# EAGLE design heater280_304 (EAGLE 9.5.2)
DATABASE: Z:\Eigene Dateien\Anwendungsdaten\Eagle\partdb\exp.txt
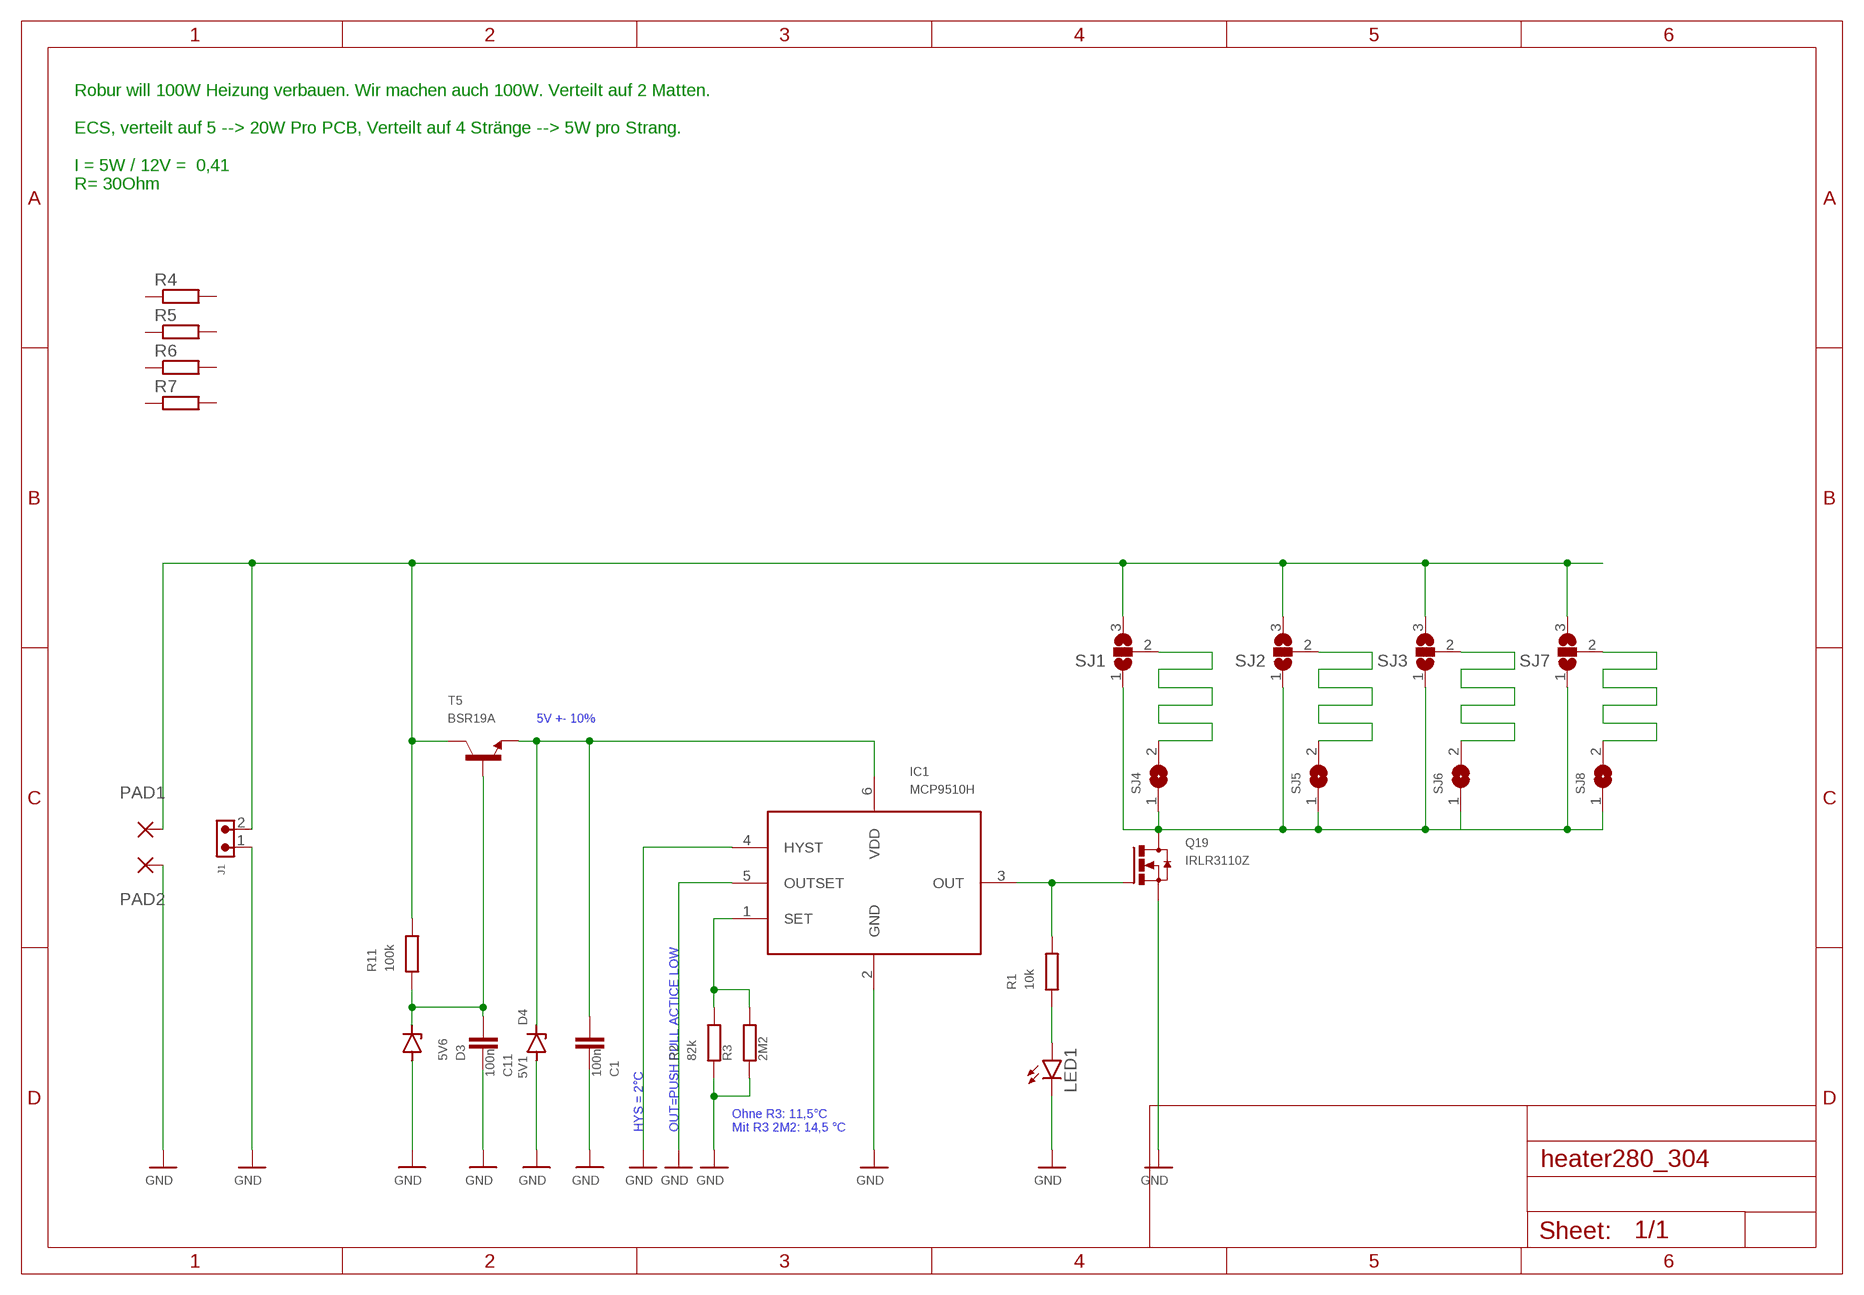
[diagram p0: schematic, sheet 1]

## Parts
C1  100n  C-EUC0603  [C0603]
C11  100n  C-EUC0603  [C0603]
D3  5V6  ZENER-DIODESOD80C  [SOD80C]
D4  5V1  ZENER-DIODESOD80C  [SOD80C]
IC1  MCP9510H  MCP9509  [SOT23-6]
J1  691322110002  [691322110002]
LED1  LEDSML0603  [SML0603]
PAD1  3,81/1,4  [3,81/1,4]
PAD2  3,81/1,4  [3,81/1,4]
Q19  IRLR3110Z  IRFR2607  [D-PACK]
R1  10k  R-EU_R0603  [R0603]
R2  82k  R-EU_R0603  [R0603]
R3  2M2  R-EU_R0603  [R0603]
R4  R-EU_R1206  [R1206]
R5  R-EU_R1206  [R1206]
R6  R-EU_R1206  [R1206]
R7  R-EU_R1206  [R1206]
R11  100k  R-EU_R0603  [R0603]
SJ1  SJ2W  [SJ_2]
SJ2  SJ2W  [SJ_2]
SJ3  SJ2W  [SJ_2]
SJ4  SJ  [SJ]
SJ5  SJ  [SJ]
SJ6  SJ  [SJ]
SJ7  SJ2W  [SJ_2]
SJ8  SJ  [SJ]
T5  BSR19A  MMBT2222ALT1-NPN-SOT23-BEC  [SOT23-BEC]

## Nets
+UB: J1.2 PAD1.1(P) R11.2 SJ1.3 SJ2.3 SJ3.3 SJ7.3 T5.C
GND: C1.2 C11.2 D3.A D4.A IC1.2(GND) IC1.4(HYST) IC1.5(OUTSET) J1.1 LED1.C PAD2.1(P) Q19.3(S) R2.1 R3.1
N$1: IC1.3(OUT) Q19.1(G) R1.2
N$2: SJ1.2 SJ4.2
N$3: C11.1 D3.C R11.1 T5.B
N$4: IC1.1(SET) R2.2 R3.2
N$5: C1.1 D4.C IC1.6(VDD) T5.E
N$6: LED1.A R1.1
N$7: SJ2.2 SJ5.2
N$8: SJ3.2 SJ6.2
N$9: SJ7.2 SJ8.2
N$11: Q19.4(D) SJ1.1 SJ2.1 SJ3.1 SJ4.1 SJ5.1 SJ6.1 SJ7.1 SJ8.1
Unconnected: R4.1 R4.2 R5.1 R5.2 R6.1 R6.2 R7.1 R7.2

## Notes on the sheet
- Robur will 100W Heizung verbauen. Wir machen auch 100W. Verteilt auf 2 Matten.
  
  ECS, verteilt auf 5 --> 20W Pro PCB, Verteilt auf 4 Stränge --> 5W pro Strang.
  
  I = 5W / 12V =  0,41
  R= 30Ohm
- 5V +- 10%
- HYS = 2°C | OUT=PUSH PULL ACTICE LOW
- Ohne R3: 11,5°C
  Mit R3 2M2: 14,5 °C

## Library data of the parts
C1 C11 = rcl:C-EU: CAPACITOR, European symbol; PARTNO: C067; SPICEPREFIX: C
D3 = diode:ZENER-DIODE: Z-Diode; PARTNO: D013
D4 = diode:ZENER-DIODE: Z-Diode; PARTNO: D012
IC1 = mcp9509:MCP9509; PARTNO: IC333
J1 = Wurth_Connectors_WR-TBL Pluggable Connector:691322110002: WR-TBL Serie 3221 - 3.50 mm Horizontal PCB Header; DATASHEET-URL: https://www.we-online.com/catalog/datasheet/691322110002.pdf; IR-UL: 10A; IR-VDE: 10.5A; MOUNT: THT; PART-NUMBER: 691322110002; PARTNO: CON212; PINS: 2; PITCH: 3.5mm; TYPE: Horizontal; WORKING-VOLTAGE-UL: 300V (AC); WORKING-VOLTAGE-VDE: 300V (AC)
LED1 = led:LED: LED; PARTNO: D078
PAD1 PAD2 = wirepad:3,81/1,4: THROUGH-HOLE PAD
Q19 = IRFR2607:IRFR2607; PARTNO: T086
R1 = rcl:R-EU_: RESISTOR, European symbol; PARTNO: R221; SPICEPREFIX: R
R2 = rcl:R-EU_: RESISTOR, European symbol; PARTNO: R243; SPICEPREFIX: R
R3 R11 = rcl:R-EU_: RESISTOR, European symbol; PARTNO: R245; SPICEPREFIX: R
R4-R7 = rcl:R-EU_: RESISTOR, European symbol; PARTNO: R493; SPICEPREFIX: R
SJ1-SJ3 SJ7 = jumper:SJ2W: SMD solder JUMPER
SJ4-SJ6 SJ8 = jumper:SJ: SMD solder JUMPER
T5 = transistor-neu-to92:*-NPN-: NPN Transistror; PARTNO: T056

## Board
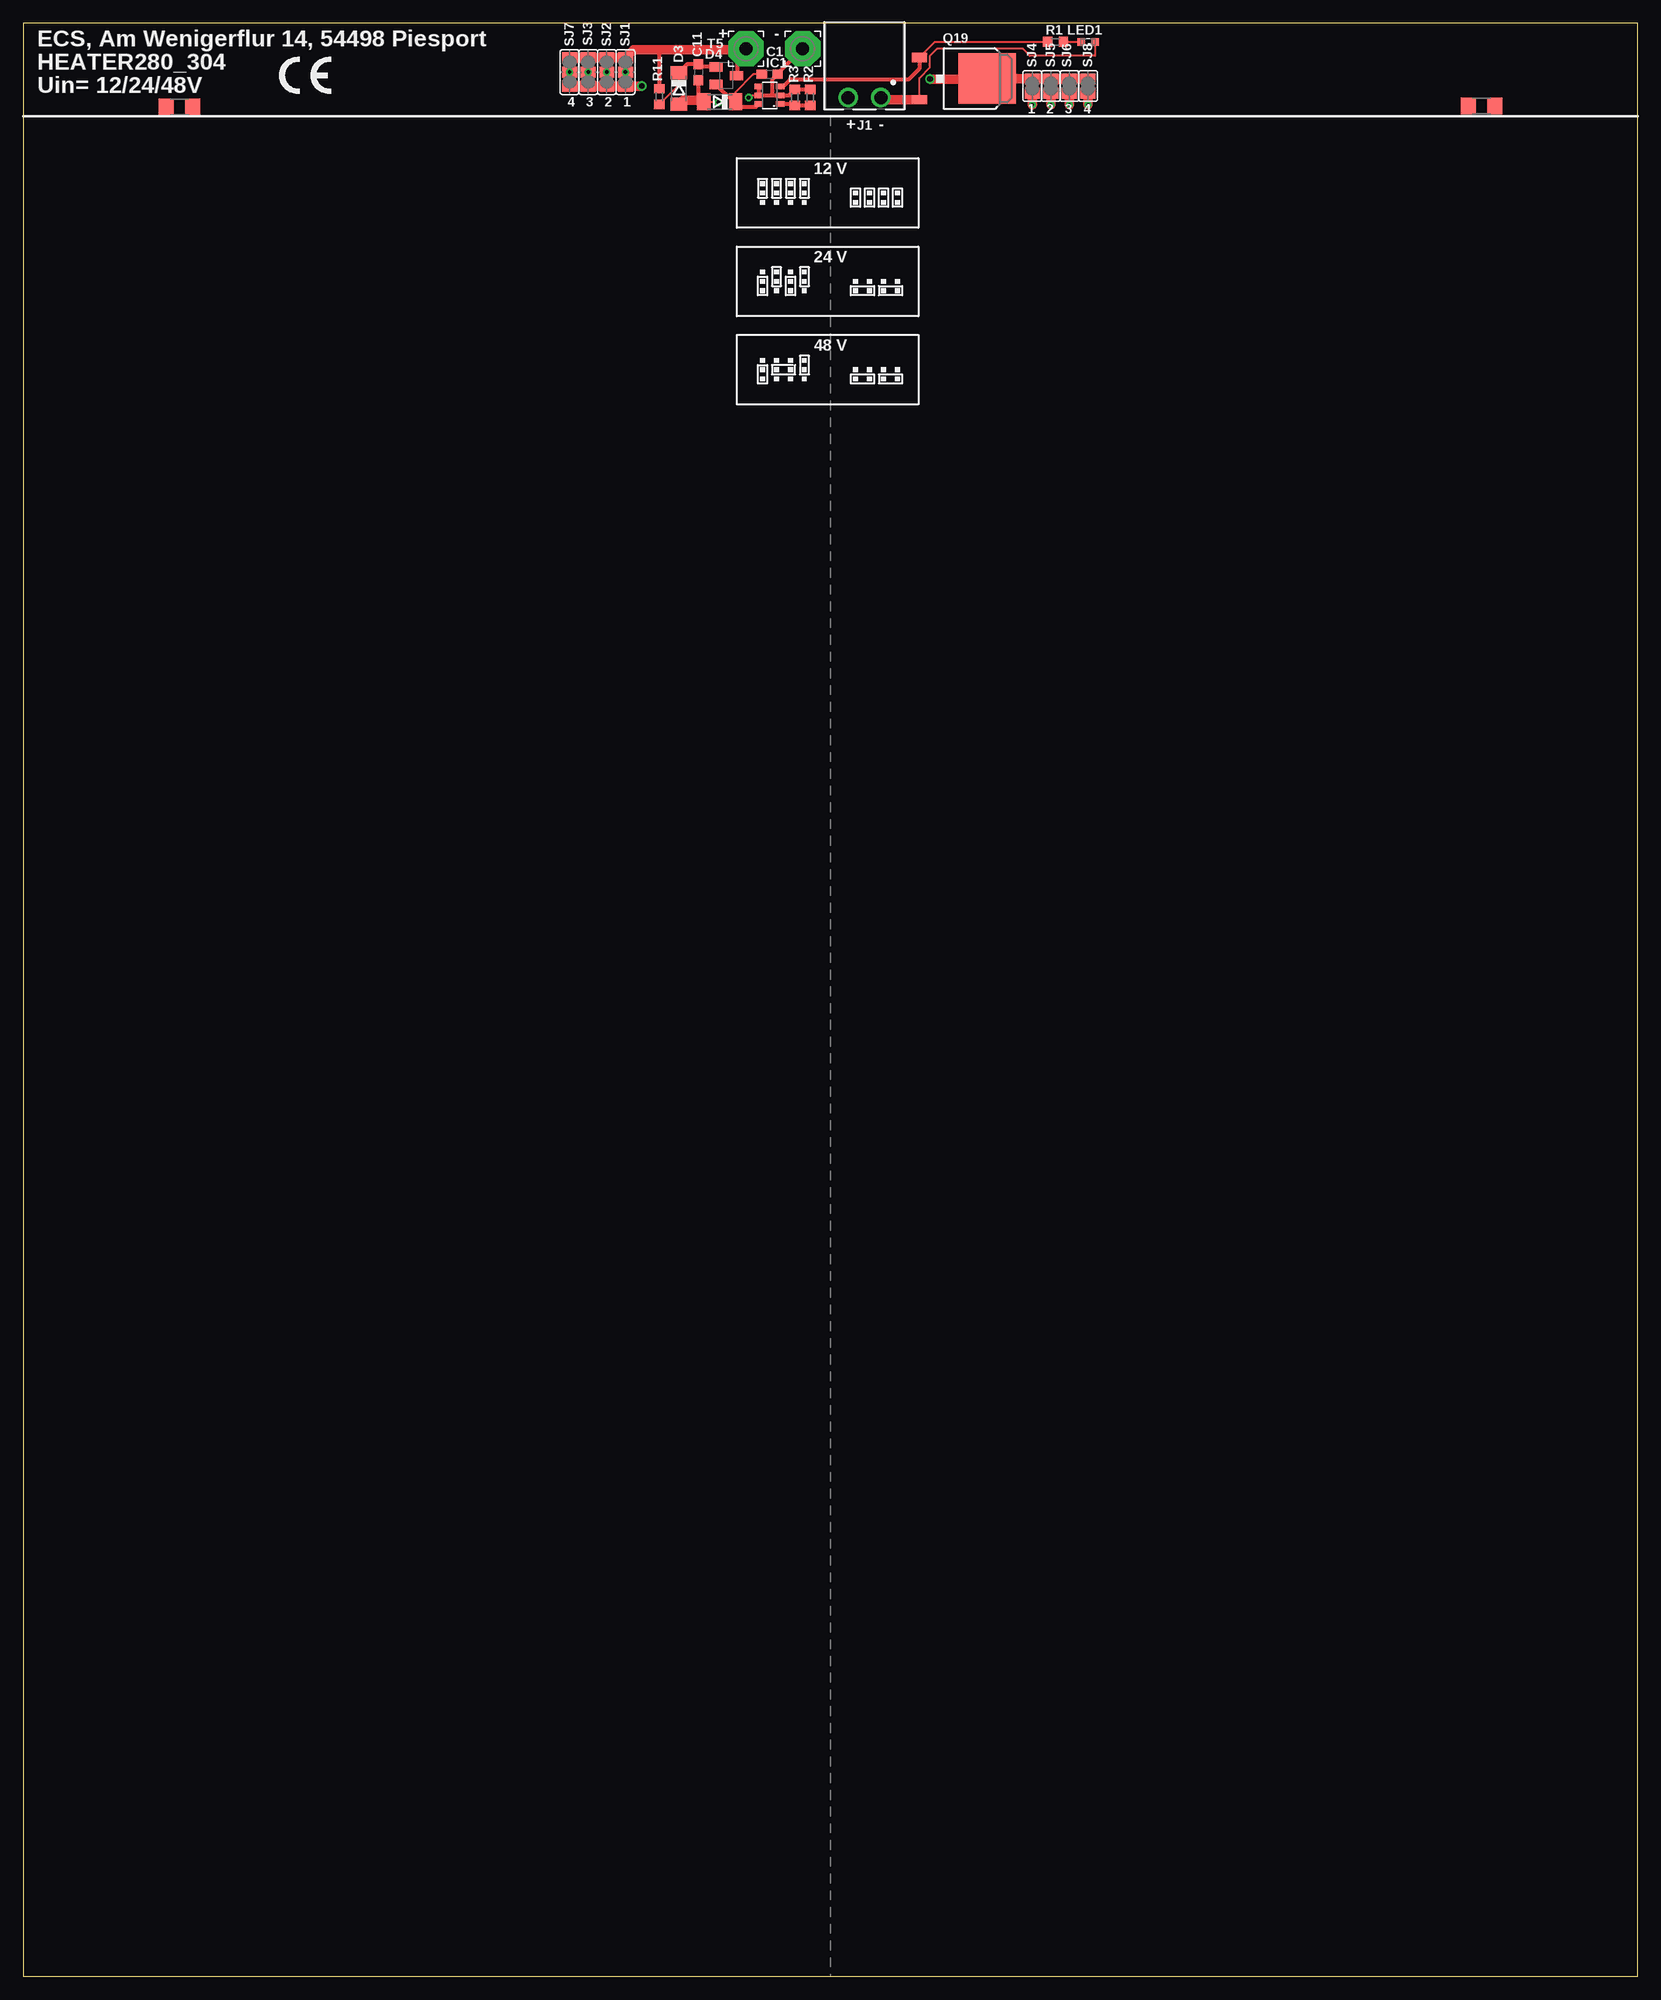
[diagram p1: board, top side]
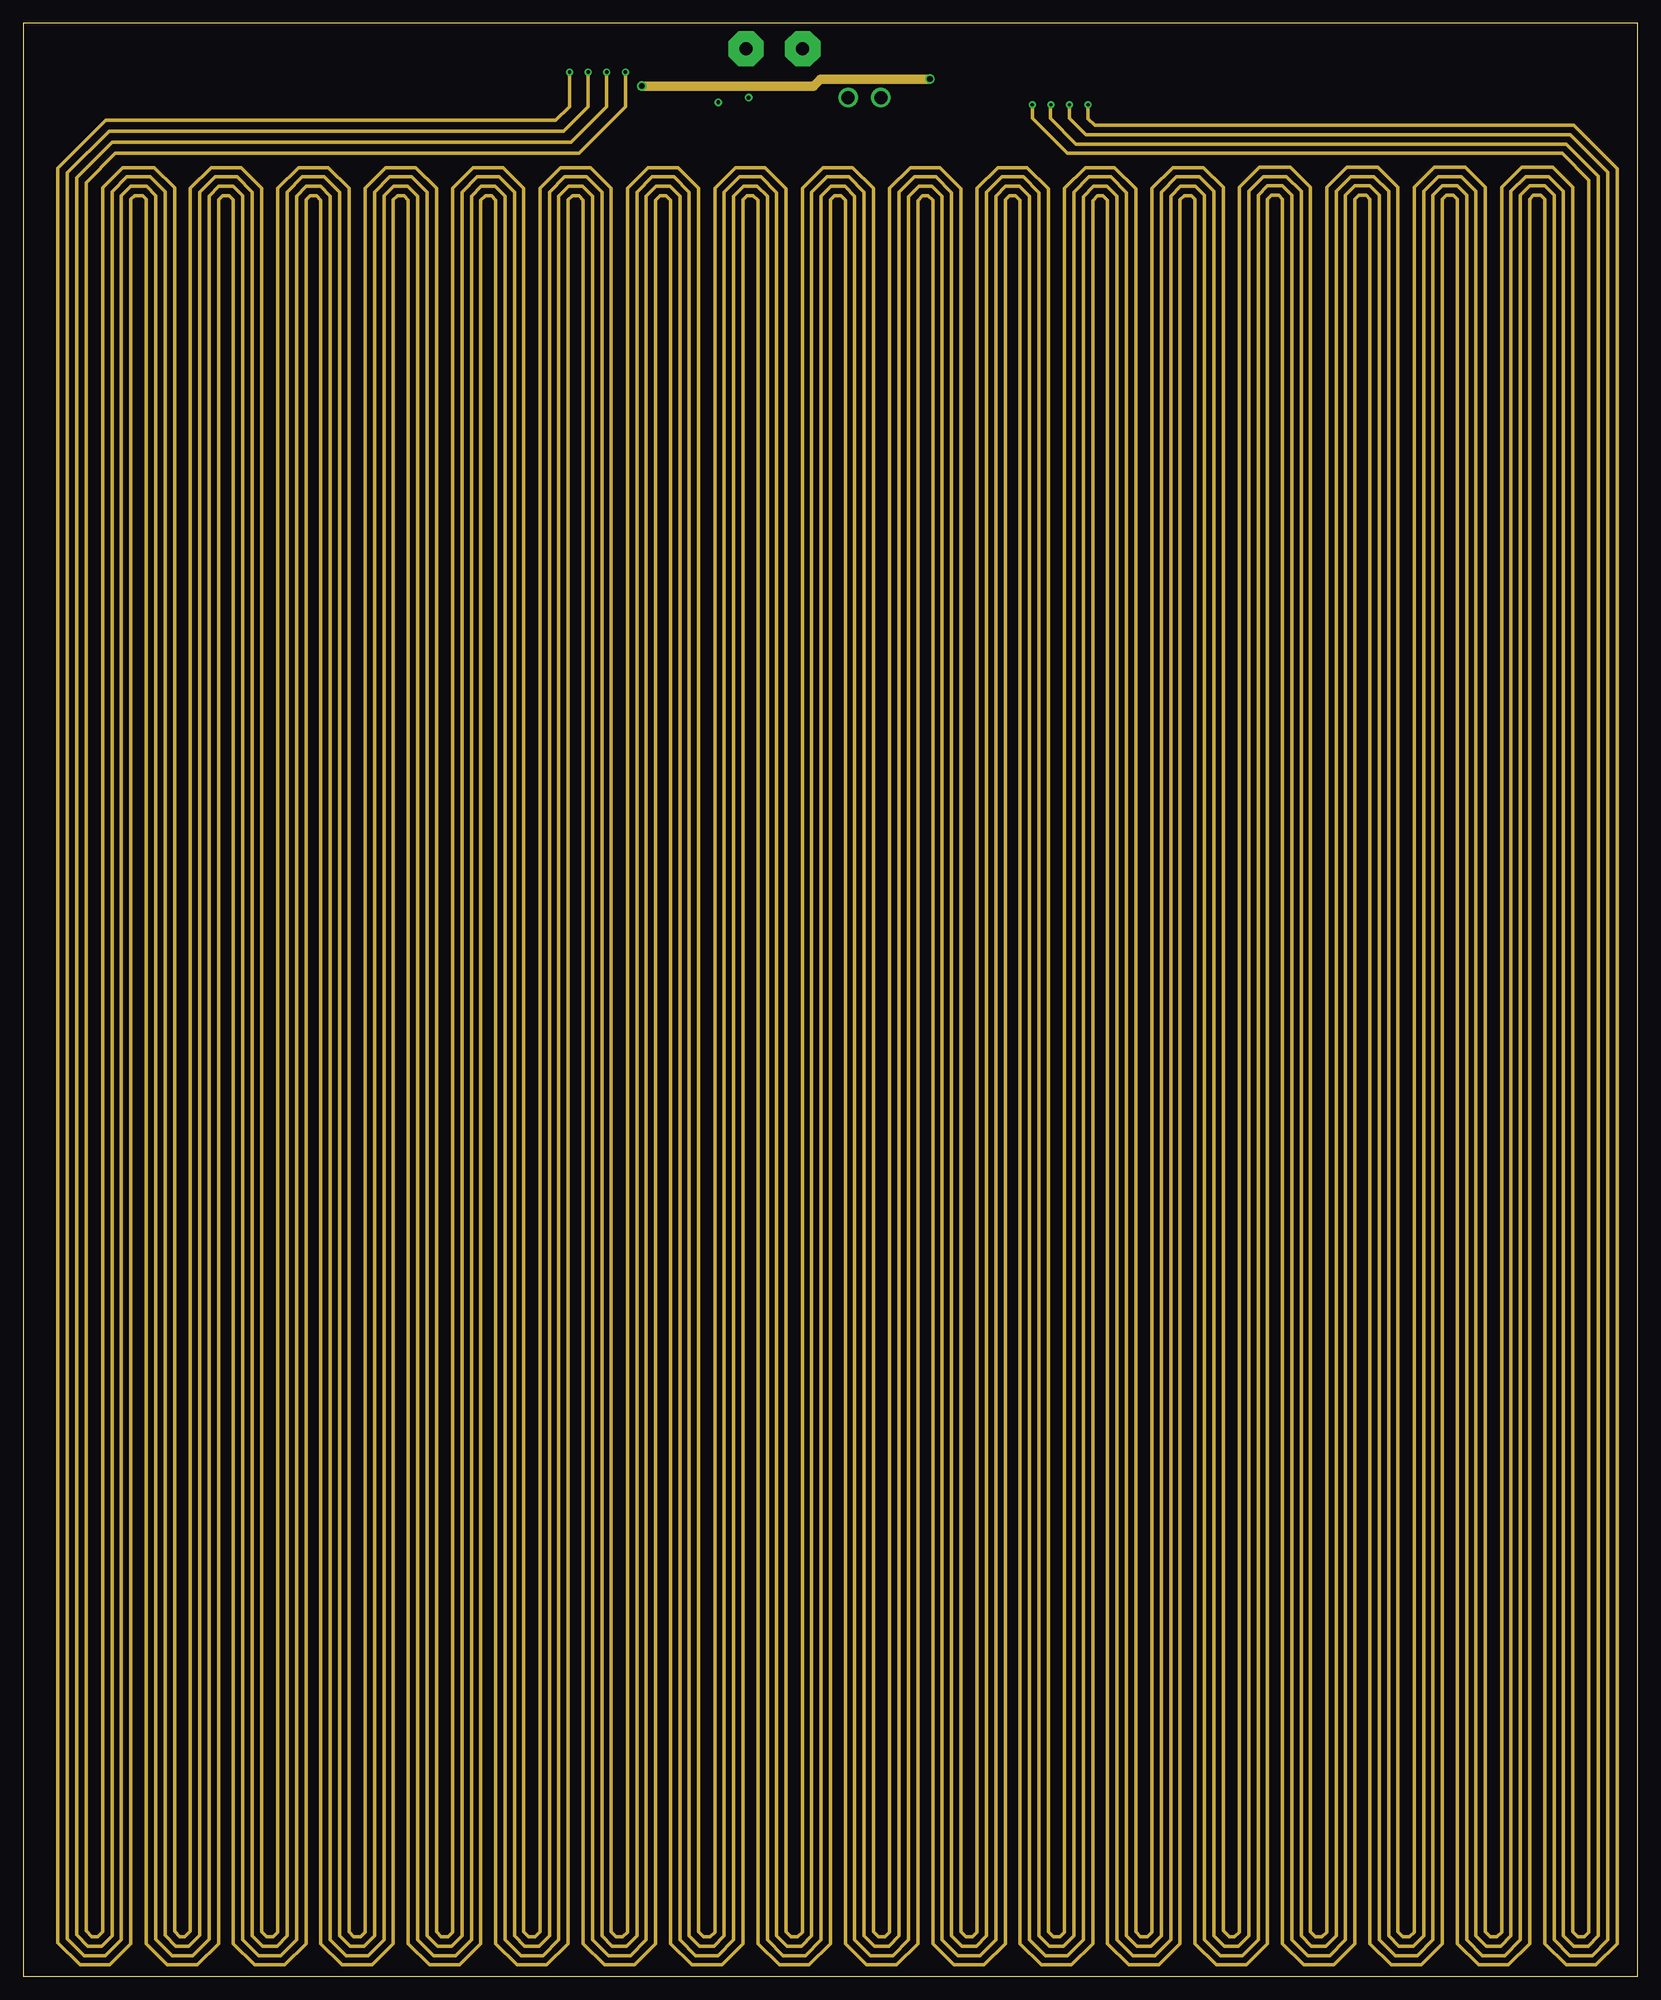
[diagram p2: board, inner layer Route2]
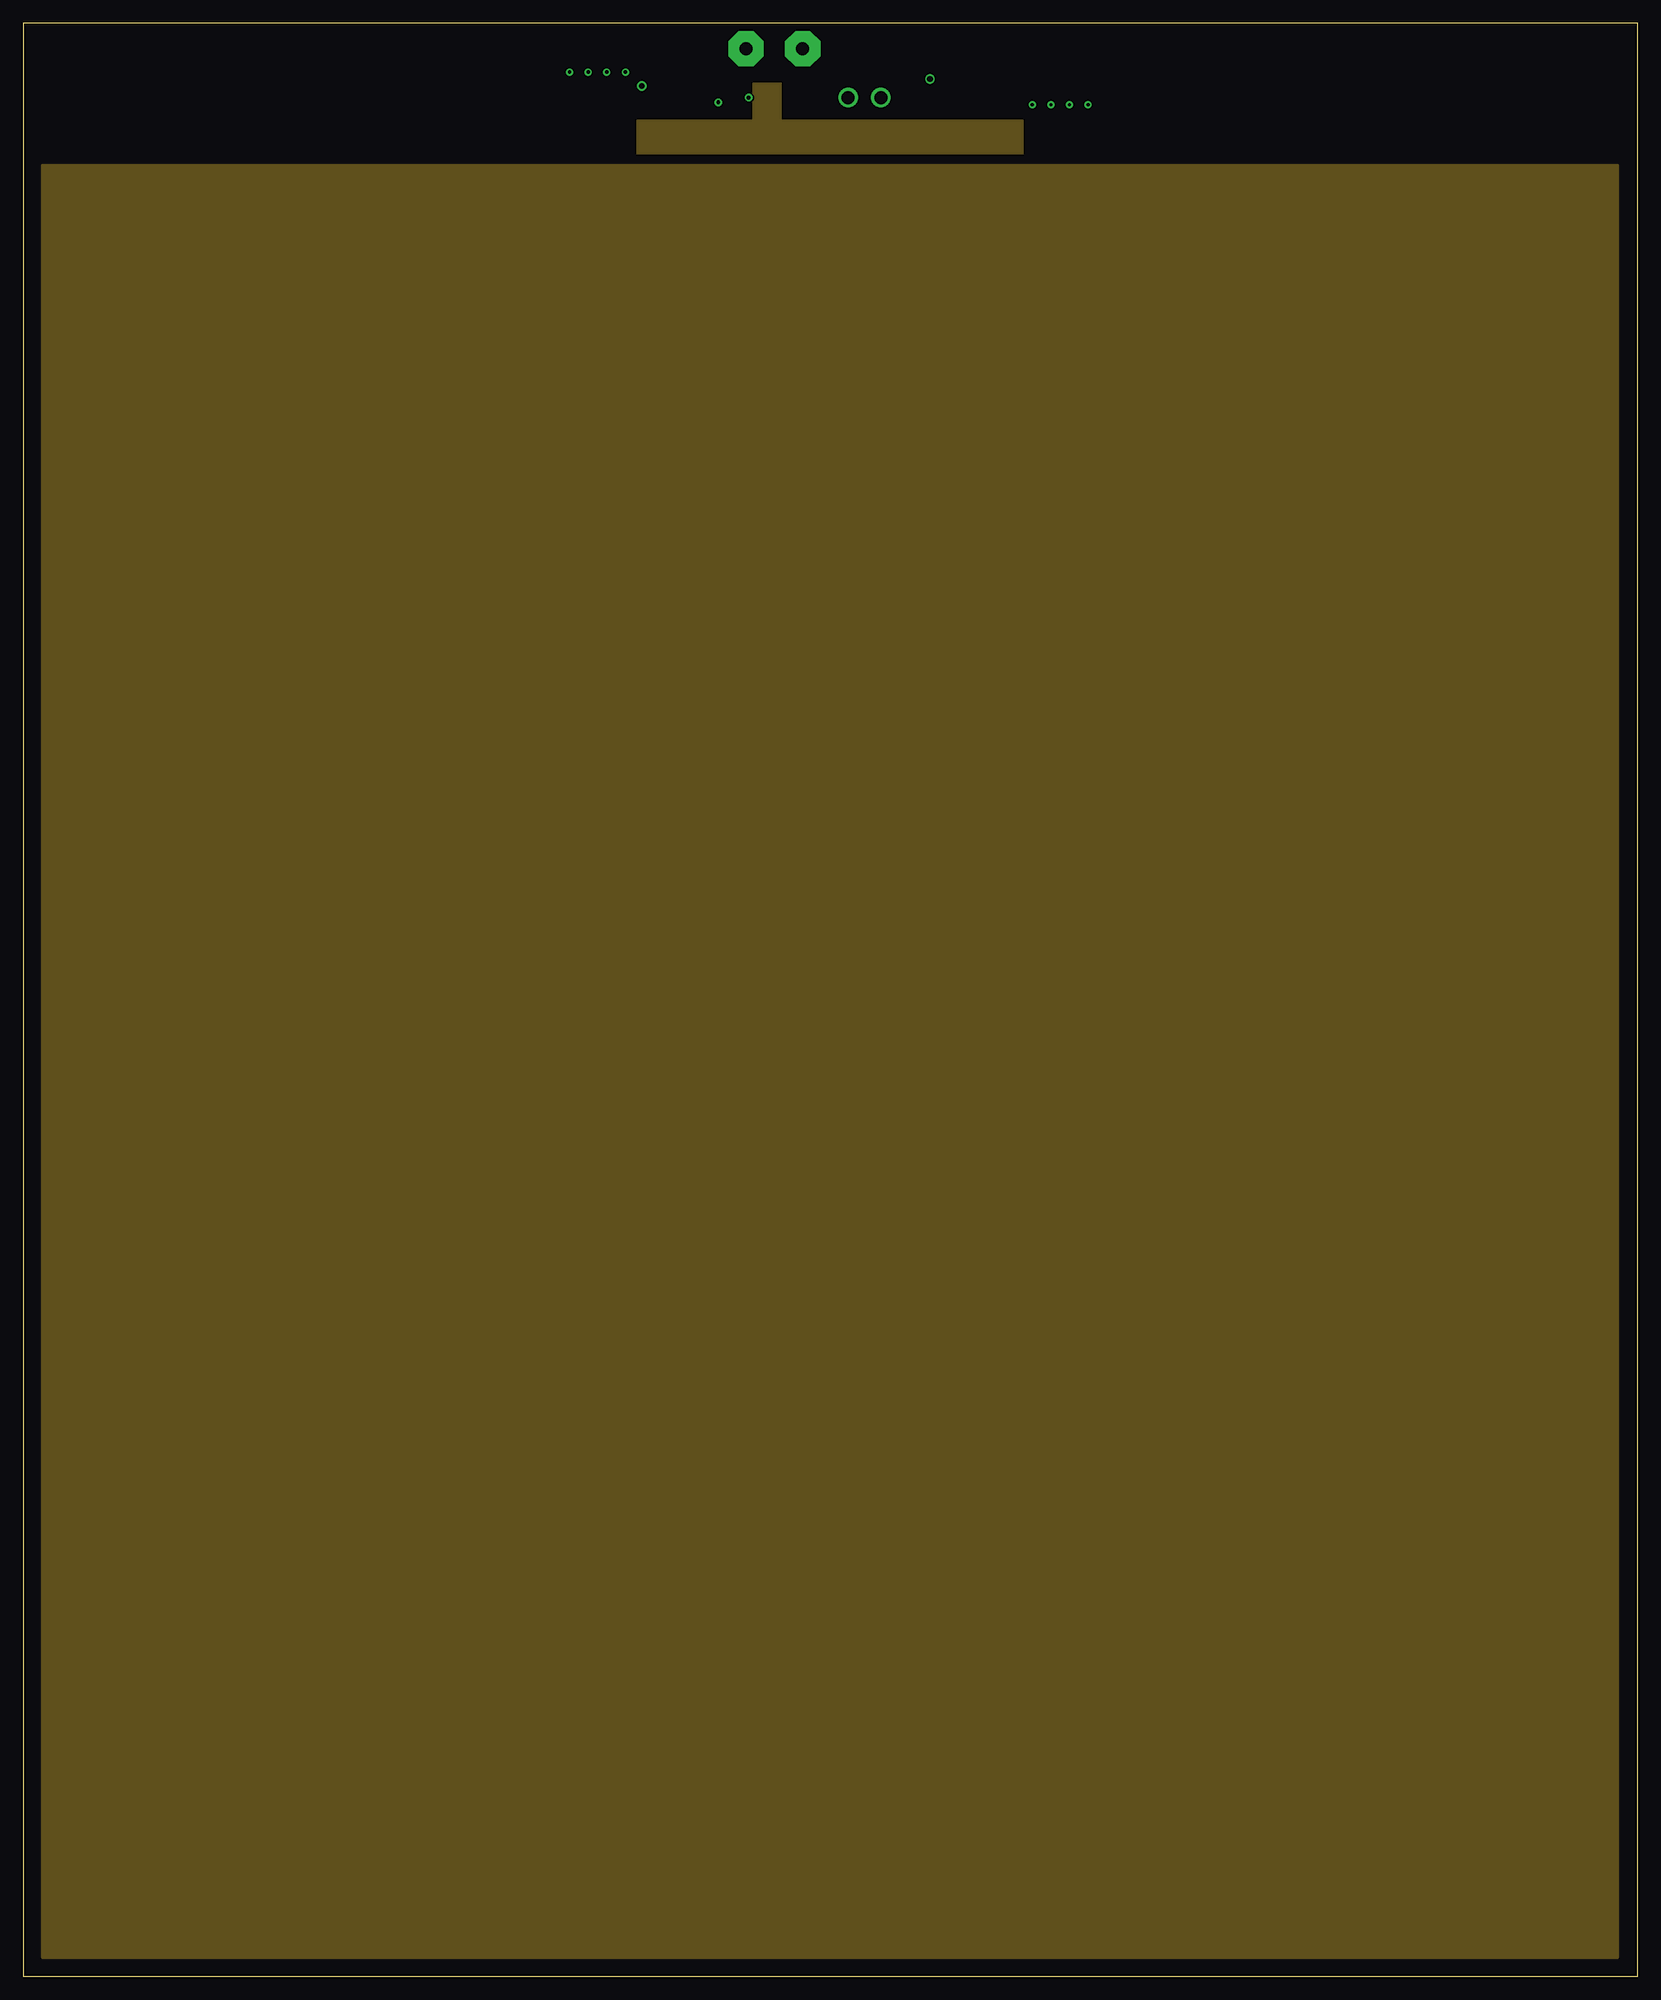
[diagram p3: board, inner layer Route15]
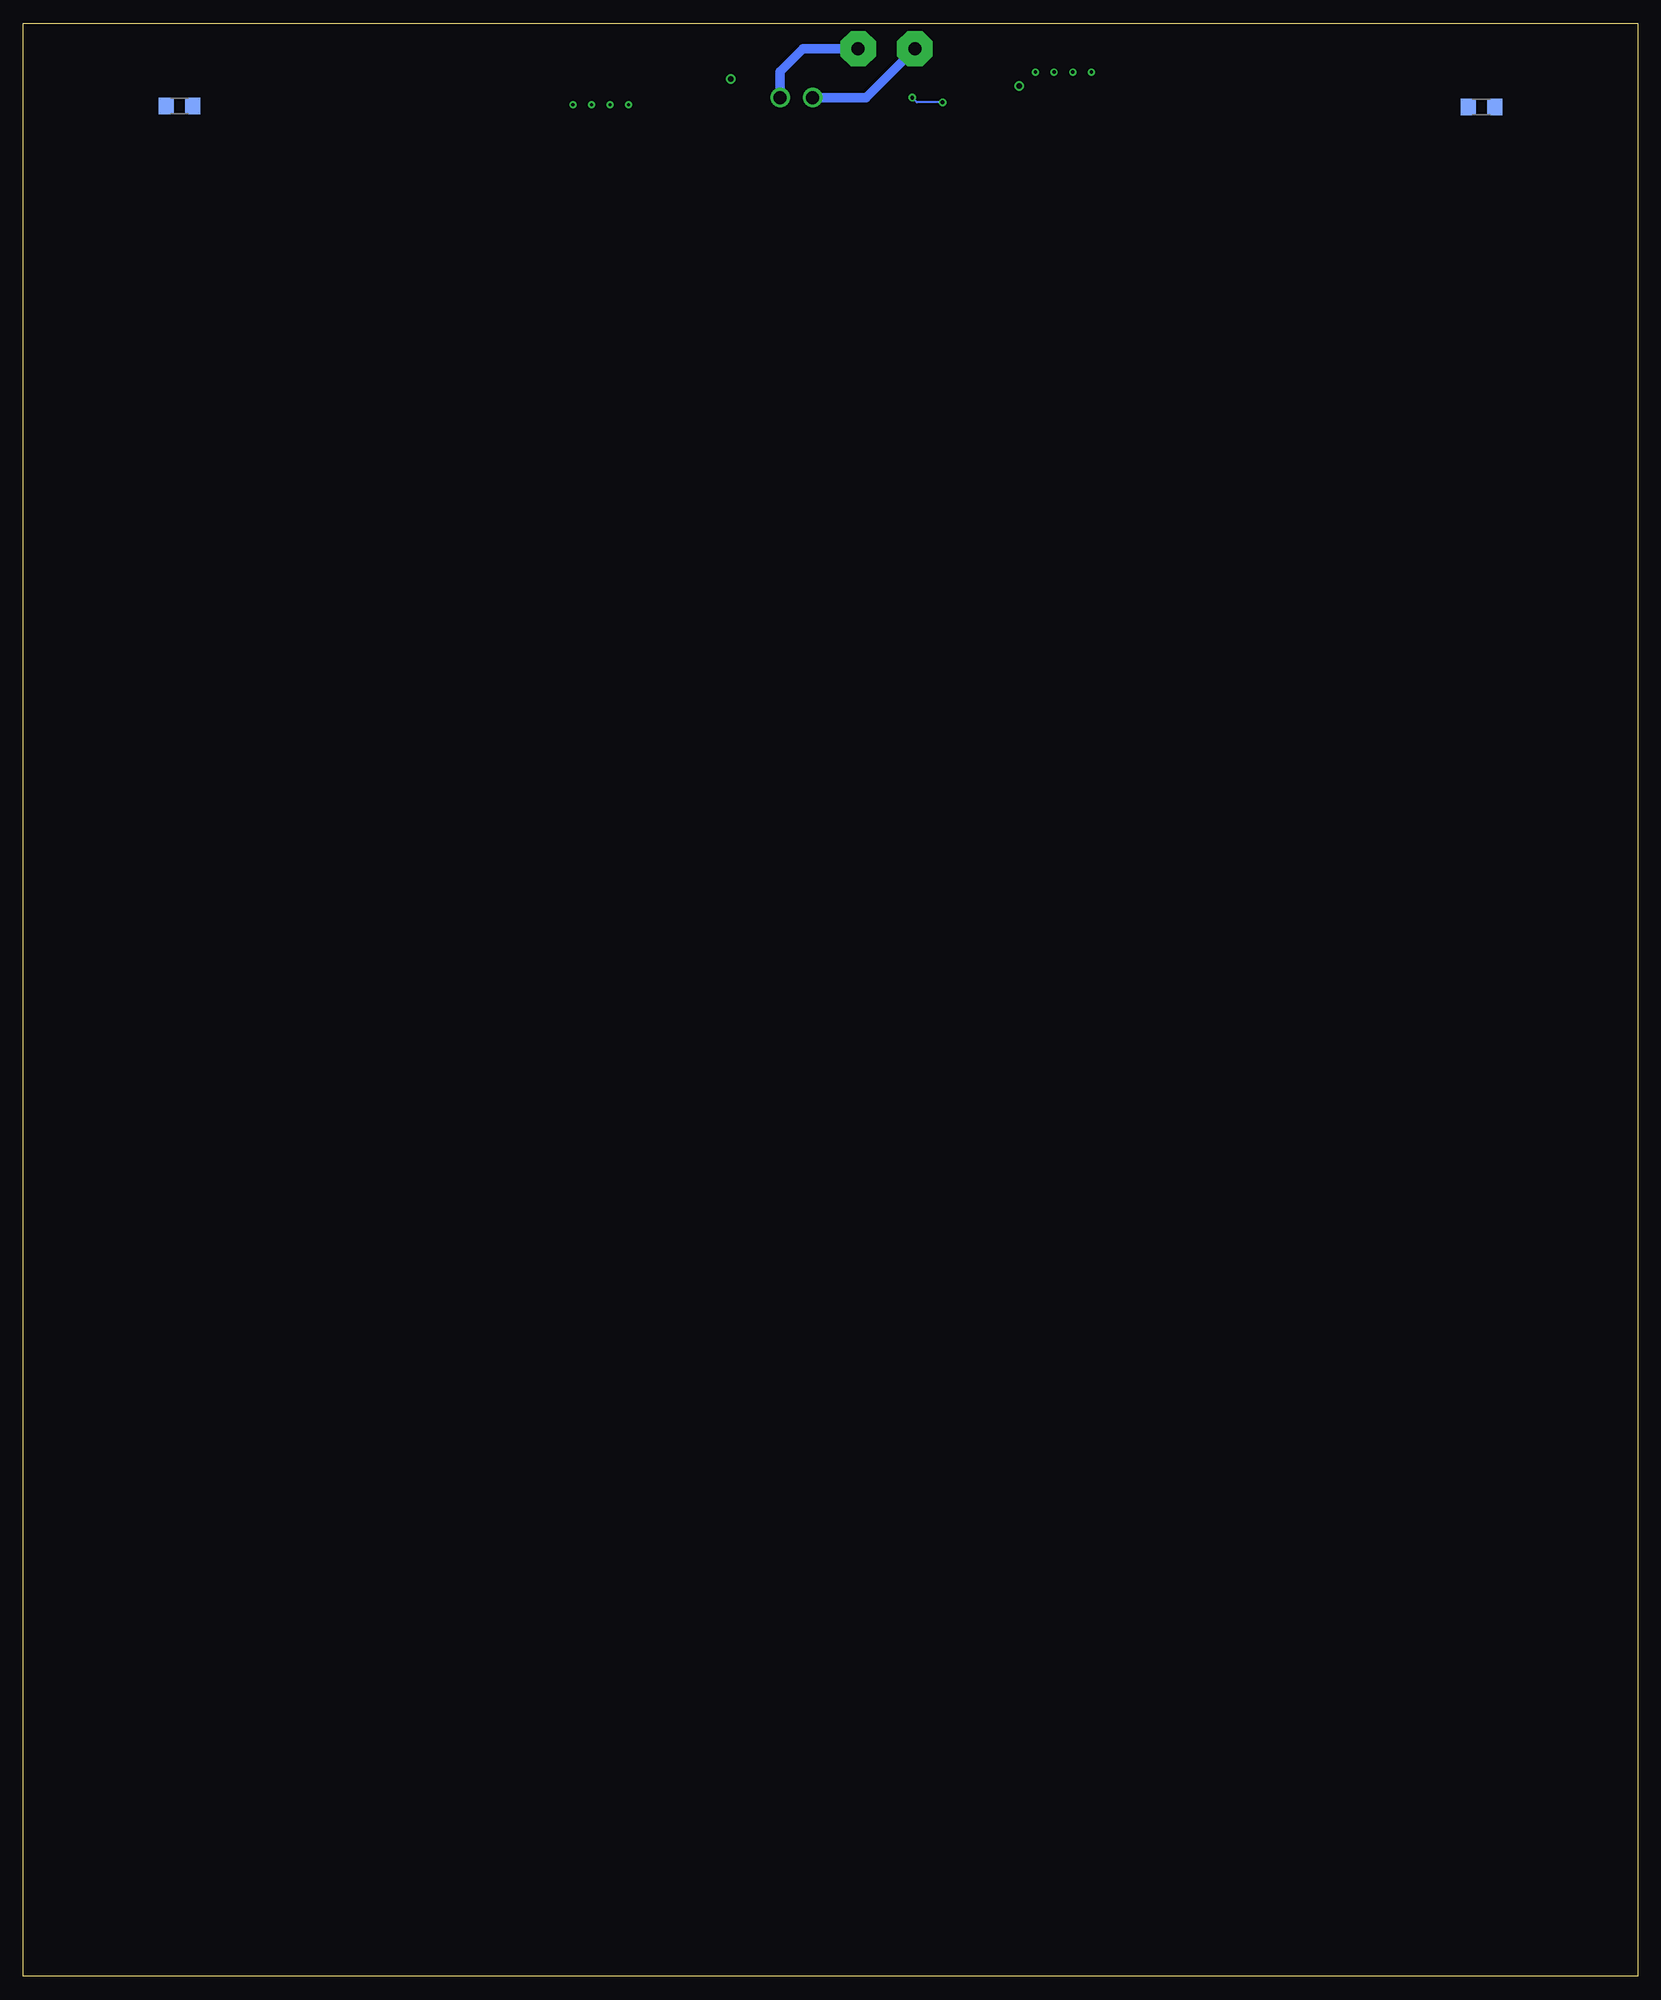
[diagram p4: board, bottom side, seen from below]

Size 173.6 x 210 mm. Coordinates in mm from the lower left corner, seen from the top.
Outline: 0,0 173.6,0 173.6,210 0,210 0,0
Copper layers (1+2*15+16): Top 0.035mm / dielectric 1.5mm / Route2 0.0175mm / dielectric 0.15mm / Route15 0.0175mm / dielectric 0.2mm / Bottom 0.035mm
Design rules "default *": minimum track width 6mil, minimum drill 0.35mm, track to track 6mil, track to pad 6mil, pad to pad 6mil, via to via 6mil, smd to smd 6mil, copper to edge 40mil, drill to drill 6mil, minimum pad ring 10mil, minimum via ring 8mil, stop-mask expansion 4mil, vias tented up to drill 0mil, thermal gap 10mil

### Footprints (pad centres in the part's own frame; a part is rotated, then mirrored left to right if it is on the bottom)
C0603 = smd 1.1 x 1: 1 -0.85,0; 2 0.85,0
SOD80C = smd 1.4 x 1.8: A 1.7,0; C -1.7,0
SOT23-6 = smd 0.6 x 0.9: 1 -0.95,-1.15; 2 0,-1.15; 3 0.95,-1.15; 4 0.95,1.15; 5 0,1.15; 6 -0.95,1.15
691322110002 = drill 1.4: 1 -1.75,0; 2 1.75,0
SML0603 = smd 0.8 x 0.8: A 0.75,0; C -0.75,0
3,81/1,4 = drill 1.397 pad 3.81 octagon: 1 0,0
D-PACK = smd 1 x 1.6: 1 -2.28,-4.8; 3 2.28,-4.8 | smd 5.4 x 6.2: 4 0,2.5
R0603 = smd 1 x 1.1: 1 -0.85,0; 2 0.85,0
R1206 = smd 1.6 x 1.803: 1 -1.422,0; 2 1.422,0
SJ_2 = smd 1.168 x 1.6: 1 -1.524,0; 2 0,0; 3 1.524,0
SJ = smd 1.168 x 1.6: 1 -0.762,0; 2 0.762,0
SOT23-BEC = smd 1 x 1.4: B -0.95,-1.1; C 0,1.1; E 0.95,-1.1

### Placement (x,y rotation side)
C1  80.27,204.52 0 top
C11  72.6,204.73 270 top
D3  70.5,203 270 top
D4  74.88,201.55 180 top
IC1  80.25,202.25 90 top
J1  90.46,202.01 180 top
LED1  114.5,208 180 top
PAD1  77.72,207.26 0 top
PAD2  83.82,207.26 0 top
Q19  101.16,204.05 270 top
R1  111,208 180 top
R2  84.64,202.02 270 top
R3  82.97,202.02 270 top
R4  16.8,201 180 top
R5  16.8,201 0 bottom
R6  156.8,201.1 0 top
R7  156.8,201.1 0 bottom
R11  68.4,202.12 90 top
SJ1  64.75,204.75 90 top
SJ2  62.75,204.75 90 top
SJ3  60.75,204.75 90 top
SJ4  108.5,203.25 270 top
SJ5  110.5,203.25 270 top
SJ6  112.5,203.25 270 top
SJ7  58.75,204.75 90 top
SJ8  114.5,203.25 270 top
T5  75.61,204.36 270 top
U$1  [CE-4MM]  27.5,202.38 0 top

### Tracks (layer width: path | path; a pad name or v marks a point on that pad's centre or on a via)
+UB
  Top 0.406: T5.C 76.75,204.4 76.75,206.29 77.61,207.15 PAD1.1 | R11.2 68.4,207.04 68.5,207.15
  Top 1.016: SJ7.3 SJ3.3 SJ2.3 SJ1.3 65.62,207.15 68.5,207.15 77.61,207.15
  Bottom 1.016: PAD1.1 82.97,202.01 J1.2
GND  (via drill 0.4)
  Top 0.2: LED1.C 115.25,206.5 108.25,206.5 107.5,207.25 98.25,207.25 97.5,206.5 97.5,205.25 96.36,204.11 Q19.3 | D4.A 74.7,201.55 v74.75,201.5 | v78,202 78.25,202.25 IC1.5
  Top 0.406: D4.A 72.6,202.13 C11.2 | 80.56,202.25 IC1.2 82.35,202.25 R3.1 R2.1 | 80.56,202.25 80.56,203.96 C1.2 81.12,204.56 PAD2.1 | IC1.4 IC1.5 80.56,202.25
  Top 1.016: D3.A 70.95,201.75 72.98,201.75 D4.A | Q19.3 92.45,201.77 J1.1
  Bottom 0.2: v74.75,201.5 77.5,201.5 v78,202
  Bottom 1.016: J1.1 92.21,204.79 89.74,207.26 PAD2.1
N$1
  Top 0.2: Q19.1 98.03,208 R1.2
  Top 0.406: IC1.3 81.7,203.2 82.5,204 95.25,204 96.36,205.11 Q19.1
N$2  (via drill 0.35, 0.35 pad 0.21)
  Top 1.016: SJ4.2 v108.5,201.25
  Route2 0.4: SJ1.2 64.75,201.02 59.79,196 9.9,196 6.75,192.85 6.75,4.87 7.37,4.26 8.01,4.26 8.54,4.78 8.54,192.32 10.71,194.49 14.09,194.49 16.26,192.32 16.26,4.82 16.84,4.25 17.38,4.25 17.97,4.84 17.97,192.26 20.2,194.49 23.41,194.49 25.63,192.27 25.63,4.77 26.16,4.25 26.86,4.25 27.37,4.75 27.37,192.26 29.6,194.49 32.79,194.49 35.03,192.25 35.03,4.77 35.55,4.25 36.26,4.25 36.77,4.75 36.77,192.27 38.99,194.49 42.19,194.49 44.43,192.25 44.43,4.77 44.95,4.25 45.66,4.25 46.17,4.75 46.17,192.26 48.4,194.49 51.59,194.49 53.83,192.25 53.83,4.77 54.35,4.25 55.05,4.25 55.35,4.55 55.57,4.77 55.57,192.26 57.8,194.49 60.99,194.49 63.23,192.25 63.23,4.77 63.75,4.25 64.47,4.25 64.97,4.75 64.97,192.26 67.2,194.49 70.39,194.49 72.63,192.25 72.63,4.77 73.16,4.25 73.86,4.25 74.37,4.75 74.37,192.26 76.6,194.49 79.75,194.49 82.03,192.22 82.03,4.77 82.56,4.25 83.26,4.25 83.77,4.75 83.77,192.26 86,194.49 89.19,194.49 91.43,192.25 91.43,4.77 91.95,4.25 92.66,4.25 93.17,4.75 93.17,192.26 95.4,194.49 98.56,194.49 100.83,192.22 100.83,4.77 101.35,4.25 102.07,4.25 102.57,4.75 102.57,192.26 104.8,194.49 107.95,194.49 110.23,192.22 110.23,4.77 110.75,4.25 111.46,4.25 111.97,4.75 111.97,192.26 114.2,194.49 117.36,194.49 119.63,192.22 119.63,4.77 120.16,4.25 120.86,4.25 121.37,4.75 121.37,192.26 123.6,194.49 126.89,194.49 129.03,192.35 129.03,4.92 129.7,4.25 130.26,4.25 130.77,4.75 130.77,192.35 132.94,194.53 136.25,194.53 138.43,192.35 138.43,4.77 138.96,4.25 139.66,4.25 140.17,4.75 140.17,192.35 142.34,194.53 145.66,194.53 147.83,192.35 147.83,4.77 148.35,4.25 149.06,4.25 149.57,4.75 149.57,192.35 151.75,194.53 155.06,194.53 157.23,192.35 157.23,4.77 157.75,4.25 158.46,4.25 158.97,4.75 158.97,192.35 161.15,194.53 164.46,194.53 166.63,192.35 166.63,4.77 167.16,4.25 167.86,4.25 168.37,4.75 168.37,193.13 165.5,196 112.3,196 108.5,199.8 v108.5,201.25
  other vias: 64.75,204.75
N$3
  Top 0.2: R11.1 70.5,203.37 D3.C
  Top 0.406: D3.C 71.38,205.58 C11.1 72.87,205.31 T5.B
N$4
  Top 0.406: IC1.1 82.97,201.3 R3.2 R2.2
N$5
  Top 0.2: C1.1 79.4,204.5 78.5,204.5 76.58,202.58 D4.C
  Top 0.406: T5.E 76.37,201.55 D4.C 76.83,201.3 76.95,201.3 77.25,201 78.77,201 IC1.6
N$6
  Top 0.2: R1.1 LED1.A
N$7  (via drill 0.35, 0.35 pad 0.21)
  Top 1.016: SJ5.2 v110.5,201.25
  Route2 0.4: SJ2.2 62.75,201.05 58.9,197.2 9.56,197.2 5.74,193.39 5.74,4.45 6.95,3.25 8.43,3.25 9.54,4.36 9.54,191.9 11.13,193.48 13.67,193.48 15.26,191.9 15.26,4.4 16.42,3.23 17.8,3.23 18.98,4.42 18.98,191.84 20.62,193.48 22.99,193.48 24.62,191.85 24.62,4.35 25.74,3.23 27.28,3.23 28.38,4.34 28.38,191.84 30.02,193.48 32.38,193.48 34.02,191.84 34.02,4.35 35.14,3.24 36.68,3.24 37.78,4.34 37.78,191.85 39.41,193.48 41.77,193.48 43.42,191.84 43.42,4.35 44.54,3.23 46.08,3.23 47.18,4.34 47.18,191.84 48.82,193.48 51.17,193.48 52.82,191.84 52.82,4.35 53.93,3.23 55.47,3.23 56.12,3.88 56.58,4.35 56.58,191.84 58.22,193.48 60.57,193.48 62.22,191.84 62.22,4.35 63.34,3.23 64.88,3.23 65.98,4.34 65.98,191.84 67.62,193.48 69.97,193.48 71.62,191.84 71.62,4.35 72.74,3.23 74.28,3.23 75.38,4.34 75.38,191.84 77.02,193.48 79.34,193.48 81.02,191.8 81.02,4.35 82.14,3.23 83.68,3.23 84.78,4.34 84.78,191.84 86.42,193.48 88.77,193.48 90.42,191.84 90.42,4.35 91.54,3.23 93.08,3.23 94.18,4.34 94.18,191.84 95.82,193.48 98.14,193.48 99.82,191.8 99.82,4.35 100.94,3.23 102.48,3.23 103.58,4.34 103.58,191.84 105.22,193.48 107.54,193.48 109.22,191.8 109.22,4.35 110.34,3.23 111.88,3.23 112.98,4.34 112.98,191.84 114.62,193.48 116.94,193.48 118.62,191.8 118.62,4.35 119.74,3.23 121.28,3.23 122.38,4.34 122.38,191.84 124.02,193.48 126.47,193.48 128.02,191.94 128.02,4.35 129.14,3.23 130.68,3.23 131.78,4.34 131.78,191.94 133.36,193.52 135.84,193.52 137.42,191.94 137.42,4.35 138.54,3.23 140.08,3.23 141.18,4.34 141.18,191.94 142.76,193.52 145.24,193.52 146.82,191.94 146.82,4.35 147.94,3.23 149.48,3.23 150.58,4.34 150.58,191.94 152.16,193.52 154.64,193.52 156.22,191.94 156.22,4.35 157.34,3.23 158.88,3.23 159.98,4.34 159.98,191.94 161.56,193.52 164.04,193.52 165.62,191.94 165.62,4.35 166.74,3.23 168.28,3.23 169.38,4.34 169.38,193.55 165.92,197.01 113.22,197.01 110.46,199.76 110.46,201.21 v110.5,201.25
  other vias: 62.75,204.75
N$8  (via drill 0.35, 0.35 pad 0.21)
  Top 1.016: SJ6.2 v112.5,201.25
  Route2 0.4: SJ3.2 60.75,201.05 58.1,198.4 9.23,198.4 4.74,193.91 4.74,4.03 6.54,2.23 8.84,2.23 10.55,3.94 10.55,191.48 11.54,192.47 13.26,192.47 14.24,191.48 14.24,3.98 16,2.23 18.22,2.23 19.99,4 19.99,191.43 21.04,192.47 22.57,192.47 23.61,191.44 23.61,3.93 25.32,2.23 27.7,2.23 29.39,3.92 29.39,191.43 30.43,192.47 31.96,192.47 33.01,191.42 33.01,3.93 34.72,2.23 37.1,2.23 38.79,3.92 38.79,191.44 39.83,192.47 41.36,192.47 42.41,191.42 42.41,3.93 44.12,2.23 46.5,2.23 48.19,3.92 48.19,191.43 49.24,192.47 50.76,192.47 51.81,191.42 51.81,3.93 53.52,2.23 55.88,2.23 57.59,3.93 57.59,191.43 58.64,192.47 60.16,192.47 61.21,191.42 61.21,3.93 62.92,2.23 65.3,2.23 66.99,3.92 66.99,191.43 68.04,192.47 69.56,192.47 70.61,191.42 70.61,3.93 72.32,2.23 74.7,2.23 76.39,3.92 76.39,191.43 77.44,192.47 78.92,192.47 80.01,191.38 80.01,3.93 81.72,2.23 84.1,2.23 85.79,3.92 85.79,191.43 86.84,192.47 88.36,192.47 89.41,191.42 89.41,3.93 91.12,2.23 93.5,2.23 95.19,3.92 95.19,191.36 96.3,192.47 97.72,192.47 98.81,191.38 98.81,3.93 100.52,2.23 102.9,2.23 104.59,3.92 104.59,191.43 105.64,192.47 107.12,192.47 108.21,191.38 108.21,3.93 109.92,2.23 112.3,2.23 113.99,3.92 113.99,191.36 115.1,192.47 116.52,192.47 117.61,191.38 117.61,3.93 119.32,2.23 121.7,2.23 123.39,3.92 123.39,191.43 124.44,192.47 126.06,192.47 127.01,191.52 127.01,3.93 128.72,2.23 131.1,2.23 132.79,3.92 132.79,191.52 133.78,192.51 135.42,192.51 136.41,191.52 136.41,3.93 138.12,2.23 140.5,2.23 142.19,3.92 142.19,191.52 143.18,192.51 144.82,192.51 145.81,191.52 145.81,3.93 147.52,2.23 149.9,2.23 151.59,3.92 151.59,191.52 152.58,192.51 154.22,192.51 155.21,191.52 155.21,3.93 156.92,2.23 159.3,2.23 160.99,3.92 160.99,191.52 161.98,192.51 163.62,192.51 164.61,191.52 164.61,3.93 166.32,2.23 168.7,2.23 170.39,3.92 170.39,193.97 166.34,198.02 114.28,198.02 112.5,199.8 v112.5,201.25
  other vias: 60.75,204.75
N$9  (via drill 0.35, 0.35 pad 0.21)
  Top 1.016: SJ8.2 v114.5,201.25
  Route2 0.4: SJ7.2 58.75,201.05 57.25,199.55 8.85,199.55 3.73,194.43 3.73,3.62 6.12,1.22 9.29,1.22 11.56,3.49 11.56,191.06 11.96,191.46 12.84,191.46 13.24,191.06 13.24,3.48 15.5,1.22 18.72,1.22 21,3.5 21,191.01 21.45,191.45 22.16,191.45 22.6,191.02 22.6,3.52 24.9,1.22 28.12,1.22 30.4,3.5 30.4,191.01 30.85,191.45 31.55,191.45 32,191 32,3.52 34.3,1.22 37.52,1.22 39.8,3.5 39.8,191.02 40.24,191.46 40.94,191.46 41.4,191 41.4,3.52 43.7,1.22 46.92,1.22 49.2,3.5 49.2,190.96 49.7,191.46 50.34,191.46 50.8,191 50.8,3.5 53.1,1.22 56.3,1.22 58.6,3.5 58.6,191.01 59.05,191.45 59.75,191.45 60.2,191 60.2,3.52 62.5,1.22 65.72,1.22 68,3.5 68,190.96 68.5,191.46 69.14,191.46 69.6,191 69.6,3.52 71.9,1.22 75.12,1.22 77.4,3.5 77.4,191.01 77.86,191.46 78.5,191.46 79,190.96 79,3.52 81.3,1.22 84.52,1.22 86.8,3.5 86.8,191.01 87.25,191.46 87.94,191.46 88.4,191 88.4,3.52 90.7,1.22 93.92,1.22 96.2,3.5 96.2,190.94 96.72,191.46 97.3,191.46 97.8,190.96 97.8,3.52 100.1,1.22 103.32,1.22 105.6,3.5 105.6,191.01 106.06,191.46 106.7,191.46 107.2,190.96 107.2,3.52 109.5,1.22 112.72,1.22 115,3.5 115,190.94 115.52,191.46 116.1,191.46 116.6,190.96 116.6,3.52 118.9,1.22 122.12,1.22 124.4,3.5 124.4,191.01 124.86,191.46 125.64,191.46 126,191.1 126,3.52 128.3,1.22 131.52,1.22 133.8,3.5 133.8,191.1 134.2,191.5 135,191.5 135.4,191.1 135.4,3.52 137.7,1.22 140.92,1.22 143.2,3.5 143.2,191.1 143.6,191.5 144.4,191.5 144.8,191.1 144.8,3.52 147.1,1.22 150.32,1.22 152.6,3.5 152.6,191.1 153,191.5 153.8,191.5 154.2,191.1 154.2,3.52 156.5,1.22 159.72,1.22 162,3.5 162,191.1 162.4,191.5 163.2,191.5 163.6,191.1 163.6,3.52 165.9,1.22 169.12,1.22 171.4,3.5 171.4,194.38 166.75,199.03 115.22,199.03 114.5,199.75 v114.5,201.25
  other vias: 58.75,204.75
N$10
  pour Route15: 78.5,203.5 78.5,199.5 66,199.5 66,196 107.5,196 107.5,199.5 105.5,199.5 81.5,199.5 81.5,203.5
N$11  (via drill 0.6)
  Top 1.016: SJ7.1 SJ3.1 SJ2.1 SJ1.1 66.48,203.23 v66.5,203.25 | SJ8.1 SJ6.1 SJ5.1 SJ4.1 104.65,204.01 103.66,205 Q19.4 103.61,204 v97.5,204
  Route2 1.016: v66.5,203.25 85,203.25 85.75,204 v97.5,204
N$12
  pour Route15: 66,194.75 2,194.75 2,194.5 2,2 171.5,2 171.5,194.75

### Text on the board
tPlace: ECS, Am Wenigerflur 14, 54498 Piesport | + | - | HEATER280_304 | Uin= 12/24/48V | 4 | 3 | 2 | 1 | 1 | 2 | 3 | 4 | + | - | 12 V | 24 V | 48 V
